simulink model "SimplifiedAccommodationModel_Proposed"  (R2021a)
settings: Solver=FixedStepAuto  StartTime=0.0  StopTime=10  FixedStep=0.00005  RelTol=1e-3  EnableMultiTasking=on
model workspace (MAT data in the model file):
  AccomRange : Simulink.Parameter (value not decoded)
  FastIntegGain : Simulink.Parameter (value not decoded)
  FastIntegTimeConstant : Simulink.Parameter (value not decoded)
  MotorLatency : Simulink.Parameter (value not decoded)
  NeuralBias : Simulink.Parameter (value not decoded)
  NeuralMyopia : Simulink.Parameter (value not decoded)
  PlantTimeConstant : Simulink.Parameter (value not decoded)
  RefractiveError : Simulink.Parameter (value not decoded)
  SensoryLatency : Simulink.Parameter (value not decoded)
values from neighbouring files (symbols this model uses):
  AccomRange = 6    [PlotSignalsForHyperopePlusLens.m]    (also in PlotACAratio.m = 2; PlotACAratioCycloplegia.m = 10; PlotACAratioCycloplegiaPresbyope.m = 1; PlotNearpointCycloplegia.m = 10)
  NeuralBias = getVariable(workspace,'NeuralBias')    [PlotNearpointCycloplegia.m]    (also in PlotSignalsForMyope.m; PlotOcularPowerCycloplegia.m)
  RefractiveError = 0    [PlotSignalsForEmmetropePlusLens.m]    (also in PlotSignalsForMyope.m = 2)
symbols that are objects in the model workspace (value not decoded): FastIntegGain, FastIntegTimeConstant, MotorLatency, NeuralMyopia, PlantTimeConstant, SensoryLatency

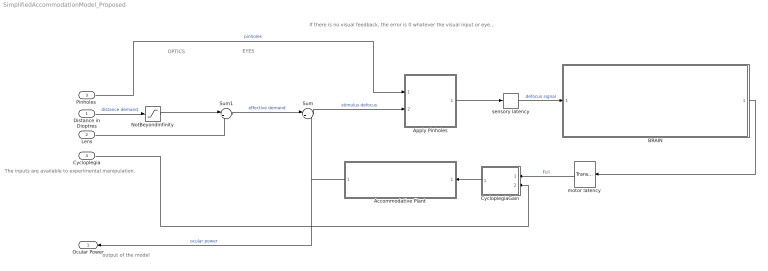
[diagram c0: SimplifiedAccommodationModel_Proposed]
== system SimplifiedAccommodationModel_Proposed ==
  note: output of the model
  note: The inputs are available to experimental manipulation.
  note: OPTICS
  note: EYES
  note: If there is no visual feedback, the error is 0 whatever the visual input or eye state
  Distance in Dioptres : Inport
  Lens : Inport  Port=2
  "Pinholes " : Inport  Port=3
  Cycloplegia : Inport  Port=4
  Accommodative Plant : Subsystem
  Apply Pinholes : MATLAB Function  TreatAsAtomicUnit=on
  BRAIN : Subsystem  Description=|
      | Accommodation system. 
      | It receives 3 inputs:
      | 1) Accommodative demand
      | 2) Convergence accommodation tonic signal
      | 3) Convergence accommodation phasic signal
      | 
      | It provides 3 outputs:
      | 1) The accommodation of the lens
      | 2) Accommodative convergence tonic signal
      | 2) Accommodative convergence phasic signal
  CycloplegiaGain : MATLAB Function  TreatAsAtomicUnit=on
  NotBeyondInfinity : Saturate  UpperLimit=100  LowerLimit=0
  Sum : Sum  Inputs=|+-  InputSameDT=on  SaturateOnIntegerOverflow=on
  Sum1 : Sum  Inputs=|+-
  motor latency : TransportDelay  DelayTime=MotorLatency
  sensory latency : TransportDelay  DelayTime=SensoryLatency
  Ocular Power : Outport
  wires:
  Distance in Dioptres/1 -> NotBeyondInfinity/1  "distance demand"
  Sum/1 -> Apply Pinholes/2(demand)  "stimulus defocus"
  Lens/1 -> Sum1/2
  Sum1/1 -> Sum/1  "effective demand"
  "Pinholes "/1 -> Apply Pinholes/1(pinholesON)  "pinholes"
  NotBeyondInfinity/1 -> Sum1/1
  Accommodative Plant/1(Ocular power) -> Sum/2, Ocular Power/1  "ocular power"
  Apply Pinholes/1(y) -> sensory latency/1
  sensory latency/1 -> BRAIN/1(Retinal defocus)  "defocus signal"
  motor latency/1 -> CycloplegiaGain/1(signal)  "Fcil"
  CycloplegiaGain/1(output) -> Accommodative Plant/1(Ciliary muscle input)
  Cycloplegia/1 -> CycloplegiaGain/2(drug)
  BRAIN/1(Oculomotor nerve signal) -> motor latency/1

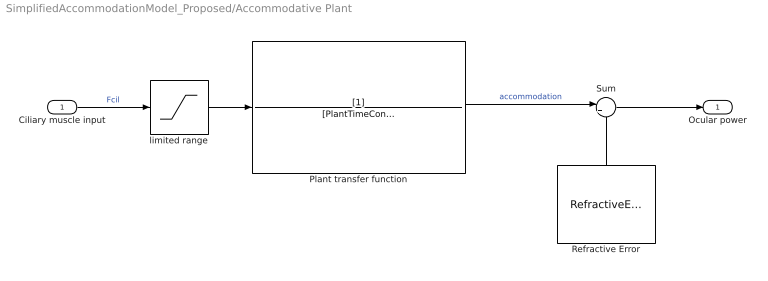
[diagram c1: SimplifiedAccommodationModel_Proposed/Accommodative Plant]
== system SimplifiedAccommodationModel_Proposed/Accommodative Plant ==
  Ciliary muscle input : Inport
  Plant transfer function : TransferFcn  Denominator=[PlantTimeConstant 1]
  Refractive Error : Constant  Value=RefractiveError
  Sum : Sum  Inputs=|++
  limited range : Saturate  UpperLimit=AccomRange  LowerLimit=0
  Ocular power : Outport
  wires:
  Ciliary muscle input/1 -> limited range/1  "Fcil"
  Refractive Error/1 -> Sum/2
  Sum/1 -> Ocular power/1
  Plant transfer function/1 -> Sum/1  "accommodation"
  limited range/1 -> Plant transfer function/1

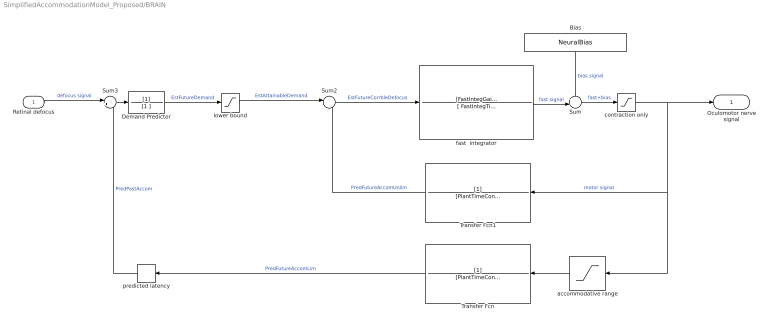
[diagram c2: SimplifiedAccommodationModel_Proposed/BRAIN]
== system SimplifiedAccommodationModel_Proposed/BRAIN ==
  Retinal defocus : Inport
  Bias : Constant  Value=NeuralBias
  Demand Predictor : TransferFcn  Denominator=[1 ]
  Sum : Sum  Inputs=++|
  Sum2 : Sum  Inputs=|+-
  Sum3 : Sum  Inputs=|++
  Transfer Fcn : TransferFcn  Denominator=[PlantTimeConstant 1]
  Transfer Fcn1 : TransferFcn  Denominator=[PlantTimeConstant 1]
  accommodative range : Saturate  UpperLimit=AccomRange  LowerLimit=0
  contraction only : Saturate  UpperLimit=Inf  LowerLimit=NeuralMyopia
  fast  integrator : TransferFcn  Numerator=[FastIntegGain]  Denominator=[ FastIntegTimeConstant 1]
  lower bound : Saturate  UpperLimit=Inf  LowerLimit=0
  predicted latency : TransportDelay  DelayTime=SensoryLatency+MotorLatency
  Oculomotor nerve signal : Outport
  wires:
  Sum3/1 -> Demand Predictor/1
  fast  integrator/1 -> Sum/2  "fast signal"
  Sum/1 -> contraction only/1  "fast+bias"
  Retinal defocus/1 -> Sum3/1  "defocus signal"
  Demand Predictor/1 -> lower bound/1  "EstFutureDemand"
  contraction only/1 -> Transfer Fcn1/1, accommodative range/1, Oculomotor nerve signal/1  "motor signal"
  predicted latency/1 -> Sum3/2  "PredPastAccom"
  Bias/1 -> Sum/1  "bias signal"
  lower bound/1 -> Sum2/1  "EstAttainableDemand"
  Sum2/1 -> fast  integrator/1  "EstFutureCorrbleDefocus"
  Transfer Fcn/1 -> predicted latency/1  "PredFutureAccomLim"
  Transfer Fcn1/1 -> Sum2/2  "PredFutureAccomUnlim"
  accommodative range/1 -> Transfer Fcn/1

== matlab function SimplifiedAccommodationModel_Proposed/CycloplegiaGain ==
function output = fcn(signal,drug)
% Modeling cycloplegia as a gain


% Clip strength of drug to the range 0 to 1:
drug(drug<0) = 0;
drug(drug>1) = 1;
output = (1-drug)*signal;

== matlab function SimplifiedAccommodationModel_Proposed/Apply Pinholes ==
function y = fcn(pinholesON,demand)
if pinholesON>0
    y = 0;
else
    y = demand;
end
